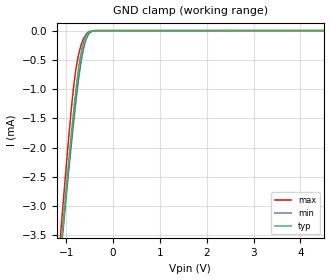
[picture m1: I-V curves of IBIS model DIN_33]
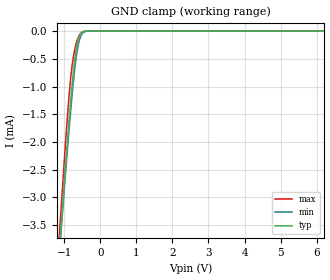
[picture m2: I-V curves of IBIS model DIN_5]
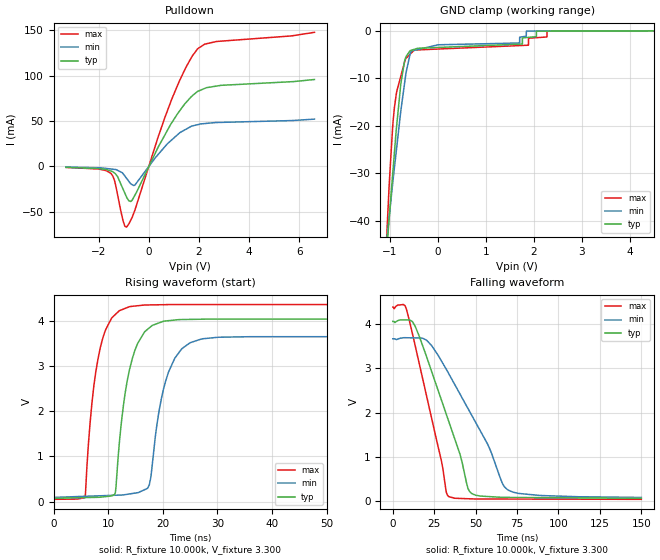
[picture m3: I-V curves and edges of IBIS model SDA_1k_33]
|Texas Instruments Incorporated
|Programmable Gamma-Voltage Generator
|   with Integrated Two-Bank Memory and External EEPROM
| Marketing part#   Digital Voltage Range   Package-type   #pins
|BUF12840RGER   2.0V to 5.5V   VQFN   24
|BUF12840RGET   2.0V to 5.5V   VQFN   24
[IBIS Ver]   4.0
[File name]   buf12840.ibs
[File Rev]   1.0
[Date]   10/09/2010
[Source]   Texas Instruments Incorporated.
   Analog-eLab, HPA
   12500 TI Blvd
   Dallas, TX -75243
   For Support e-mail: elab_ibis@list.ti.com
|   SIMDE - V2.0 201002 Build 340
[Notes]   Revision History:
   1.0: 10/09/2010
   - Initial version of the model
   - Initial Model generated from simulations in TISPICED
   - Model names with a trailing _33 contains the model for
   3.3V (3.0V and 3.6V).
   _ Model names with trailing _5 contains
   the model for 5V (4.5V and 5.5V) operation.
   - Model not matched to measurements
   - C_comp although listed in numerical order of value are
   obtained from varying PVT conditions. For PVT conditions
   for each specific value refer the buffer description under
   respective [Model]. IBIS model user is responsible for using
   appropriate C_comp to simulate for Signal Integrity.
[Disclaimer]
 This product is designed as an aid for customers of Texas Instruments.
 No warranties, either expressed or implied, with respect to this third
 party software (if any) or with respect to its fitness for any
 particular purpose is claimed by Texas Instruments or the author. The
 software (if any) is provided solely on an "as is" basis. The entire
 risk as to its quality and performance is with the customer
[Copyright] (C) Copyright 2009 Texas Instruments Incorporated.
   All rights reserved.
|   BUF12840
[Component]   buf12840rge
[Manufacturer] TI
[Package]   | 24 VQFN - RGE package
| variable   typ   min   max
R_pkg  4.67870E-02   4.13200E-02   5.41400E-02
L_pkg  1.11572E+00nH 9.63170E-01nH 1.32027E+00nH
C_pkg  1.19598E-01pF 1.11070E-01pF 1.28900E-01pF
|-------------------------PIN------------------------------------------------
[Pin] signal_name  model_name  R_pin  L_pin C_pin
1   OUT5   TERM   0.05086  1.23137nH  0.12241pF
2   OUT4   TERM   0.04516  1.07488nH  0.12017pF
3   OUT3   TERM   0.04211  0.99364nH  0.11375pF
4   OUT2   TERM   0.04196  0.98983nH  0.11343pF
5   OUT1   TERM   0.04477  1.06438nH  0.11921pF
6   OUT0   TERM   0.05028  1.21556nH  0.11835pF
7   VS   POWER   0.02966  1.15130nH  0.16878pF
8   GND_A   GND   0.02604  0.95475nH  0.16633pF
9   VSD   POWER   0.05073  1.22321nH  0.12921pF
10  EA1   DIN   0.04677  1.11491nH  0.12224pF
11  EA0   DIN   0.04541  1.07748nH  0.11899pF
12  EN   DIN   0.04801  1.14887nH  0.11473pF
13  LD   DIN   0.05080  1.22207nH  0.12047pF
14  SCL   DIN   0.04543  1.07348nH  0.11909pF
15  SDA   SDA   0.04290  1.00507nH  0.11368pF
16  A0   DIN   0.04132  0.96317nH  0.11107pF
17  BKSEL   DIN   0.04225  0.98825nH  0.11273pF
18  GND_D   GND   0.04514  1.06887nH  0.11213pF
19  OUT11   TERM   0.05365  1.30017nH  0.12890pF
20  OUT10   TERM   0.04862  1.16138nH  0.12610pF
21  OUT9   TERM   0.04612  1.09521nH  0.12101pF
22  OUT8   TERM   0.04624  1.09991nH  0.12129pF
23  OUT7   TERM   0.04894  1.17458nH  0.12680pF
24  OUT6   TERM   0.05414  1.32027nH  0.12754pF
|   Model Selectors
[Model Selector]  DIN
DIN_33   3.3V digital input
DIN_5   5V digital input
|NOTES   Model DIN split into two Models DIN_33 and DIN_5
|   to accomodate vast voltage range of 2.0V - 5.5V
|   DIN_33 operates in voltage range of 3.0 - 3.3 - 3.6
|   DIN_5 operates in voltage range of 4.5 - 5 - 5.5
|   The max pin frequency for Model DIN is 3.4MHz.Also the
|   voltage range and frequency is referenced with datasheet.
[Model Selector]  SDA
SDA_1k_33  3.3V digital output
SDA_1k_5   5V digital output
|NOTES   Model SDA split into two Models SDA_33 and SDA_5
|   to accomodate vast voltage range of 2.7V - 5.5V
|   SDA_33 operates in voltage range of 3 - 3.3 - 3.6
|   SDA_5 operates in voltage range of 4.5 - 5 - 5.5
|   The max pin frequency for Model SDA is 3.4MHz.Also the
|   voltage range and frequency is referenced with datasheet.
|   TERM Model
[Model] TERM
Model_type Terminator
C_comp   1e-20   1e-20   1e-20
| variable   typ   min   max
[Voltage Range]   3.3V   2.0V   5.5V
[POWER Clamp Reference]  3.3V   2.0V   5.5V
[GND Clamp Reference]   0.0V   0.0V   0.0V
|Operating Temperature   27   95   -40
[Temperature Range]   57   125   -40
| Models and submodels in the file (5): TERM (Terminator), DIN_33 (Input), DIN_5 (Input), SDA_1k_33 (I/O_open_drain), SDA_1k_5 (I/O_open_drain)
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|   DIN_33 Model
[Model] DIN_33
|Signals EA1(10), EA0(11), EN(12), LD(13), SCL(14), A0(16), BKSEL(17)
Model_type Input
Vinl = 0.99
Vinh = 2.31
|   typ   min   max
|   (nom PVT)   (Fast PVT)   (slow PVT)
C_comp   9.6231540e-13  9.4183370e-13  9.9743640e-13
| Where   nom PVT is  Nominal Process, 3.3V, 57C
|   Fast PVT is Strong Process, 3.6V, -40C
|   Slow PVT is Weak Process, 3.0V, 125C
[Voltage Range]   3.3   3   3.6
[Temperature Range]   57   125   -40
|Ambient Temperature   27   95   -40
[Power Clamp Reference]   3.3   3   3.6
[GND Clamp Reference]   0   0   0
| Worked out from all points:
|   GND clamp passes 1 mA (typ) near -0.79 V on its own axis
[GND Clamp]
|   Voltage   I(typ)   I(min)   I(max)
-3.3V     -25.15mA   -23.94mA   -26.88mA
-1.143V   -3.987mA   -4.061mA   -3.705mA
-1.07V    -3.317mA   -3.431mA   -2.983mA
-899.3mV  -1.831mA   -2.012mA   -1.399mA
-841.3mV  -1.371mA   -1.562mA   -947.9uA
-799.5mV  -1.061mA   -1.252mA   -689uA
-719.1mV  -549.4uA   -728.1uA   -351.2uA
-667.9mV  -317.8uA   -458.5uA   -210.2uA
-588mV    -105.5uA   -178.6uA   -80.59uA
-509.1mV  -22.78uA   -52.61uA   -14.99uA
-346.6mV  -743.3nA   -940.4nA   -1.051uA
6.6V      0A         0A         0A
[POWER Clamp]
|   SCR cell for ESD function. Effects occurr above VDD x 2
|   Voltage   I(typ)   I(min)   I(max)
-3.3V     0A         0A         0A
0V        0A         0A         0A
6.6V      0A         0A         0A
|   INPUT 5V Model
[Model]   DIN_5   |Rload to VDD = 1k ohms
Model_type   Input
|Signals EA1(10), EA0(11), EN(12), LD(13), SCL(14), A0(16), BKSEL(17)
Vinl = 1.5
Vinh = 3.5
|   typ   min   max
|   (Fast PVT)   (Nom PVT)   (slow PVT)
C_comp   9.4484000e-13  9.0543380e-13  9.4889750e-13
| Where   Nom PVT is  Nominal Process, 5.0V, 57C
|   Fast PVT is Strong Process, 5.5V, -40C
|   Slow PVT is Weak Process, 4.5V, 125C
[Voltage Range]   5   4.5   5.5
[Temperature Range]   57   125   -40
|Ambient Temperature   27   95   -40
[Power Clamp Reference]   5   4.5   5.5
[GND Clamp Reference]   0   0   0
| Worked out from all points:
|   GND clamp passes 1 mA (typ) near -0.79 V on its own axis
[GND Clamp]
|   Voltage   I(typ)   I(min)   I(max)
-5V       -42.18mA   -39.94mA   -45.76mA
-1.136V   -3.924mA   -4.002mA   -3.632mA
-1.1V     -3.586mA   -3.684mA   -3.279mA
-1.092V   -3.513mA   -3.616mA   -3.202mA
-905.9mV  -1.891mA   -2.067mA   -1.456mA
-803.4mV  -1.085mA   -1.283mA   -710.1uA
-735.7mV  -641.4uA   -831uA     -409.4uA
-677.9mV  -356.5uA   -507.2uA   -234uA
-602.5mV  -129.4uA   -216.1uA   -100.9uA
-508.9mV  -21.88uA   -52.89uA   -14.91uA
-345.8mV  -624.9nA   -912.1nA   -917.4nA
10V       0A         0A         0A
[POWER Clamp]
|   SCR cell for ESD function. Effects occurr above VDD x 2
|   Voltage   I(typ)   I(min)   I(max)
-5V       0A         0A         0A
0V        0A         0A         0A
10V       0A         0A         0A
|   SDA_33 Model
[Model] SDA_1k_33
|Signals SDA(15)
Model_type   I/O_open_drain
Polarity   Non-Inverting
Enable   Active-Low
Vinl = 0.99
Vinh = 2.31
Vmeas = 1.65
Vref = 1.65
Cref = 0pF
Rref = 10000
| Rpullup to DVDD = 1k
|   typ   min   max
|   (nom PVT)   (slow PVT)   (Fast PVT)
|   Output high impedance
|C_comp   2.0762000e-12  2.0690870e-12  2.1137920e-12
| Where   nom PVT is  Nominal Process, 3.3V, 57C
|   Fast PVT is Strong Process, 3.6V, -40C
|   Slow PVT is Weak Process, 3.0V, 125C
|   typ   min   max
|   (nom PVT)   (slow PVT)   (Fast PVT)
|   Output High
C_comp   1.4979290e-10  1.0710390e-10  2.5469060e-10
| Where   nom PVT is  Nominal Process, 3.3V, 57C
|   Fast PVT is Strong Process, 3.6V, -40C
|   Slow PVT is Weak Process, 3.0V, 125C
[Voltage Range]   3.3   3   3.6
[Temperature Range]   57   125   -40
|Ambient Temperature   27   95   -40
[Pullup Reference]   3.3   3   3.6
[Pulldown Reference]   0   -0   0
[Power Clamp Reference]   3.3   3   3.6
[GND Clamp Reference]   0   -0   -0
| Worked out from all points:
|   slope of the pulldown table from 0 to 0.495 V, typ, clamps not added: 17.9 ohm
|   falling waveform, R_fixture 10.000k, V_fixture 3.300: 20-80 % time 21.5ns typ, 29.5ns min, 15.9ns max; typ from 4.05 V to 0.071 V
|   rising waveform, R_fixture 10.000k, V_fixture 3.300: 20-80 % time 2.88ns typ, 3.25ns min, 2.57ns max; typ from 0.071 V to 4.05 V
[Pulldown]
|   Voltage   I(typ)   I(min)   I(max)
-3.3V     -972.7uA   -657.3uA   -1.057mA
-1.512V   -5.021mA   -2.805mA   -7.559mA
-1.368V   -7.157mA   -3.27mA    -15.12mA
-1.031V   -24.58mA   -7.717mA   -59.06mA
-890.8mV  -33.38mA   -12.85mA   -66.79mA
-722.2mV  -38.54mA   -19.04mA   -59.33mA
-552.8mV  -31.61mA   -20.35mA   -48.02mA
930.5mV   48.75mA    29.62mA    75.03mA
1.487V    70.44mA    41.02mA    109.4mA
1.947V    82.56mA    45.97mA    129.5mA
2.694V    88.43mA    48.34mA    137.5mA
6.6V      95.68mA    52.04mA    147.6mA
[GND Clamp]
|   Voltage   I(typ)   I(min)   I(max)
-3.3V     -371.1mA   -274.2mA   -586.1mA
-1.13V    -54.81mA   -50.07mA   -56.13mA
-1.02V    -39.86mA   -39.5mA    -33.15mA
-943.5mV  -30.16mA   -32.06mA   -20.12mA
-871.2mV  -21.08mA   -25.55mA   -13.49mA
-774.3mV  -11.19mA   -16.9mA    -9.597mA
-696.6mV  -6.463mA   -11.13mA   -6.675mA
-580mV    -4.222mA   -4.926mA   -4.992mA
1.7V      -2.864mA   -2.62mA    -3.164mA
1.848V    -1.478mA   -107uA     -3.101mA
2.279V    -127.7uA   -97.23uA   -150.7uA
6.6V      0A         0A         0A
[POWER Clamp]
|   SCR cell for ESD function. Effects occurr above VDD x 2
|   Voltage   I(typ)   I(min)   I(max)
-3.3V     0A         0A         0A
0V        0A         0A         0A
6.6V      0A         0A         0A
[Ramp]
R_load = 10000
|   typ   min   max
dV/dt_r   1.94288/2.87253e-009   1.74316/3.21422e-009   2.13391/2.56689e-009
dV/dt_f   1.94288/2.15045e-008   1.74316/2.95729e-008   2.13391/1.58573e-008
[Falling Waveform]
R_fixture = 10.000k
V_fixture = 3.300
V_fixture_min = 3.000
V_fixture_max = 3.600
C_fixture = 0.000
|  time   V(typ)   V(min)   V(max)
0s        4.052V     3.661V     4.375V
8.308ns   4.085V     3.684V     4.314V
13.58ns   3.935V     3.68V      3.491V
20.33ns   3.262V     3.63V      2.381V
29.37ns   2.278V     3.159V     908.2mV
32.29ns   1.961V     2.973V     209.3mV
33.64ns   1.814V     2.884V     113.5mV
46.18ns   231.7mV    2.037V     60.34mV
69.25ns   91.38mV    265.3mV    54.95mV
150ns     71.45mV    90.51mV    48.2mV
[Rising Waveform]
R_fixture = 10.000k
V_fixture = 3.300
V_fixture_min = 3.000
V_fixture_max = 3.600
C_fixture = 0.000
|  time   V(typ)   V(min)   V(max)
0s        71.45mV    90.51mV    48.2mV
5.757ns   86.82mV    115.2mV    85.4mV
7.719ns   92.05mV    123.6mV    2.863V
11.21ns   159.2mV    138.5mV    4.14V
13.96ns   2.949V     168.5mV    4.327V
17.54ns   3.856V     369.4mV    4.365V
19.7ns    3.984V     2.253V     4.37V
22.2ns    4.03V      3.18V      4.374V
27.07ns   4.048V     3.608V     4.374V
150ns     4.052V     3.661V     4.375V
